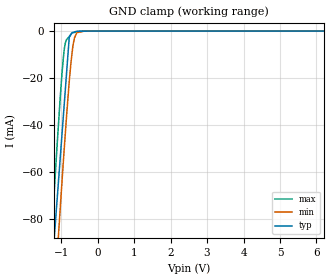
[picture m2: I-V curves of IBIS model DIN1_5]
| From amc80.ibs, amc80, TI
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[Model]  DIN1_5
Model_type   Input
Vinl = 0.8
Vinh = 2.0
|   typ   min   max
|   (nom PVT)   (Fast PVT)   (slow PVT)
C_comp   5.599E-13   5.249E-13   5.755E-13
| Where   nom PVT is  Nominal Process, 5.0V, 27C
|   Fast PVT is Strong Process, 5.5V, -40C
|   Slow PVT is Weak Process, 4.5V, 125C
|C_comp - from L-C Tank method, L = 1nH, peak frequency
[Voltage Range]   5   4.5   5.5
[Temperature Range]   27   125   -40
[Power Clamp Reference]   5   4.5   5.5
[GND Clamp Reference]   0   0   0
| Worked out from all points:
|   GND clamp passes 1 mA (typ) near -0.72 V on its own axis
[GND Clamp]
|   Voltage   I(typ)   I(min)   I(max)
-5V       -1.106A    -1.116A    -1.106A
-1.415V   -143.7mA   -172mA     -127.1mA
-1.246V   -100.3mA   -129.5mA   -83.02mA
-1.23V    -96.92mA   -125.5mA   -78.84mA
-1.127V   -75.59mA   -100.4mA   -52.97mA
-1.085V   -66.74mA   -90.01mA   -42.77mA
-930.8mV  -34.63mA   -53.93mA   -10.09mA
-777.7mV  -2.719mA   -21.62mA   -2.313mA
-699.6mV  -709.6uA   -9.376mA   -833.7uA
-570.9mV  -61.44uA   -767.5uA   -355.1uA
-355.4mV  -35.64uA   -3.928uA   -2.898uA
9.985V    0A         0A         0A
[POWER Clamp]
|   SCR cell for ESD function. Effects occurr above VDD x 2
|   Voltage   I(typ)   I(min)   I(max)
-5V       0A         0A         0A
0V        0A         0A         0A
10V       0A         0A         0A
